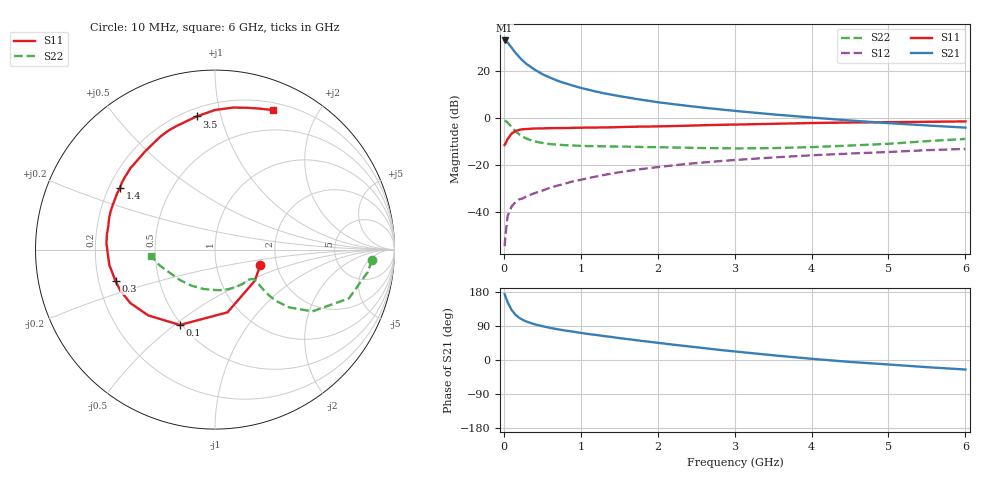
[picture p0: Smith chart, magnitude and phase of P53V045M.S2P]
! SIEMENS Small Signal Semiconductors
! BFP183
! Si NPN RF Bipolar Junction Transistor in SOT143
! VCE = 3 V  IC = 45 mA
! Common Emitter S-Parameters:  March  1996
# GHz  S  MA  R  50
!  f  S11  S21  S12  S22
! GHz  MAG  ANG  MAG  ANG  MAG  ANG  MAG  ANG
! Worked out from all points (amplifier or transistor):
!   36 points, 10 MHz to 6 GHz, reference 50 ohm
!   highest |S21| = 32.8 dB at 10 MHz (marker M1)
!   |S21| within 3 dB of that: start of sweep to 98.93 MHz
!   unconditionally stable (mu >= 1): start of sweep to 15.95 MHz; 375.4 MHz to end of sweep
!   at 250 MHz: K = 0.82, MSG = 29.1 dB, |S12| = -34.1 dB
!   at 1.4 GHz: K = 1.34, MAG = 13.3 dB, |S12| = -23.6 dB
!   at 6 GHz: K = 1.04, MAG = 3.2 dB, |S12| = -13.2 dB
!   S11 on the Smith chart (normalised r, x): 10 MHz: 1.64, -0.31; 100 MHz: 0.49, -0.52; 300 MHz: 0.27, -0.14; 1.4 GHz: 0.24, +0.28; 3.5 GHz: 0.25, +0.84; 6 GHz: 0.27, +1.47
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0.01  0.267 -19.3  43.89 174.0  0.0019 75.1  0.8757 -3.8
0.02  0.2818 -38.3  43.48 168.4  0.0031 78.4  0.8604 -8.3
0.05  0.3564 -78.7  39.69 151.9  0.0084 70.5  0.7943 -20.0
0.1  0.4634 -115.0  30.91 132.3  0.0131 55.5  0.6426 -32.4
0.15  0.5226 -135.5  24.21 119.7  0.0164 52.3  0.5245 -37.9
0.2  0.5577 -147.7  19.51 111.4  0.0187 51.8  0.4474 -40.0
0.25  0.5744 -156.3  16.14 105.4  0.0197 51.1  0.3959 -40.3
0.3  0.5812 -162.5  13.73 101.1  0.022 51.3  0.3593 -39.8
0.4  0.5947 -171.6  10.57 94.2  0.0253 54.5  0.3169 -38.6
0.5  0.5981 -178.2  8.489 89.2  0.0286 56.2  0.2933 -37.9
0.6  0.6057 176.7  7.157 84.8  0.033 57.6  0.2789 -37.5
0.7  0.6083 171.6  6.112 81.1  0.0367 59.0  0.2694 -37.7
0.8  0.6085 167.5  5.403 77.7  0.0405 59.9  0.2635 -38.3
1.1  0.6216 156.5  3.952 68.6  0.0531 60.4  0.2525 -41.7
1.4  0.631 147.2  3.103 60.8  0.0658 59.4  0.2474 -47.0
1.8  0.6546 135.9  2.409 50.2  0.0826 56.7  0.2411 -55.5
2.2  0.6711 125.7  1.96 40.5  0.0983 53.3  0.2351 -65.4
2.8  0.7114 111.6  1.52 26.7  0.1207 47.3  0.2279 -82.8
3.5  0.7488 97.9  1.186 12.5  0.1447 40.9  0.2283 -105.8
4.5  0.7975 82.8  0.88 -5.1  0.1751 31.0  0.2588 -139.1
5.5  0.8251 72.1  0.691 -18.9  0.2067 22.3  0.3209 -164.1
6  0.8424 67.3  0.622 -25.1  0.2196 17.4  0.3576 -174.5
